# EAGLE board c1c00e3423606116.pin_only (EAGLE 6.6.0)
REV: D

Size 15.24 x 26.67 mm. Coordinates in mm from the lower left corner, seen from the top.
Outline: 15.24,25.4 15.24,2.29 14.48,1.52 11.18,1.52 9.65,0 2.54,0 0.76,1.78 0,1.78 0,25.4 arc-90 1.27,26.67 4.9,26.67 5.11,26.39 10.16,26.39 10.34,26.67 13.97,26.67 arc-90 15.24,25.4
Copper layers (1*16): Top 0.035mm / dielectric 1.5mm / Bottom 0.035mm
Design rules "adafruit": minimum track width 8mil, minimum drill 15.5mil, track to track 8mil, track to pad 8mil, pad to pad 8mil, via to via 8mil, smd to smd 8mil, copper to edge 10mil, drill to drill 8mil, minimum pad ring 10mil, minimum via ring 8mil, stop-mask expansion 2mil, vias tented up to drill 20mil, thermal gap 10mil
Net classes: 1 power: width 0.305 mm
Holes 2.2 mm at 1.52,20.19 13.72,20.19

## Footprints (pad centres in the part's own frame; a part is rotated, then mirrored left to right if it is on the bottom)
CHIPLED_0805_NOOUTLINE = smd 1.2 x 1.2: A 0,-1.05; C 0,1.05
JSTPH2 = smd 1 x 4.6: 1 -1,-3.7; 2 1,-3.7 | smd 1.6 x 3.4: NC1 -3.4,1.5; NC2 3.4,1.5
0805-NO = smd 1.3 x 1.5: 1 -0.95,0; 2 0.95,0
4UCONN_20329 = smd 1 x 2: BASE@1 -0.75,-2; BASE@2 0.75,-2 | smd 0.4 x 1.35: D+ 0,0.775; D- -0.65,0.775; GND 1.3,0.775; ID 0.65,0.775; VBUS -1.3,0.775 | drill 0.7 offset: SPRT@1 -3.3,0.9; SPRT@2 3.3,0.9 | drill 0.6 pad 2.5 square: SPRT@3 -3.6,-1.9; SPRT@4 3.6,-1.9 | hole 0.7: -1.95,0; 1.95,0
1X04-CLEANBIG = drill 1.016 pad 1.778: 1 -3.81,0; 2 -1.27,0; 3 1.27,0; 4 3.81,0
SOD-323 = smd 1.35 x 0.8: A 1.27,0; C -1.27,0
SOD-123FL = smd 0.91 x 1.22: A 1.637,0; C -1.637,0
SOT23-5L = smd 0.55 x 1.2: 1 -0.95,-1.3; 2 0,-1.3; 3 0.95,-1.3; 4 0.95,1.3; 5 -0.95,1.3
1X01-CLEANBIG = drill 1.016 pad 1.778: 1 0,0
BTN_KMR2_4.6X2.8 = smd 0.9 x 1: A 2.05,0.8; A' -2.05,0.8; B 2.05,-0.8; B' -2.05,-0.8
0603-NO = smd 1.1 x 1: 1 -0.85,0; 2 0.85,0
MLF20_4X4MM_0.5MM_ATMEL = smd 0.8 x 0.25: 1 -2,1; 2 -2,0.5; 3 -2,0; 4 -2,-0.5; 5 -2,-1; 11 2,-1; 12 2,-0.5; 13 2,0; 14 2,0.5; 15 2,1 | smd 0.25 x 0.8: 6 -1,-2; 7 -0.5,-2; 8 0,-2; 9 0.5,-2; 10 1,-2; 16 1,2; 17 0.5,2; 18 0,2; 19 -0.5,2; 20 -1,2 | smd 2.6 x 2.6: THERMAL 0,0
FIDUCIAL_1MM = smd 1 x 1: 1 0,0
MOUNTINGHOLE_2.0_PLATED = drill 2.2 pad 3: P$1 0,0

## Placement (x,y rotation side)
B1  red  [CHIPLED_0805_NOOUTLINE]  13.72,24.26 0 top
BAT  JST-PH2  [JSTPH2]  7.62,23.11 0 bottom
C1  10uF  [0805-NO]  4.32,17.91 90 top
C8  10uF  [0805-NO]  10.41,3.68 270 top
CN1  microUSB  [4UCONN_20329]  7.62,22.35 180 top
CN3  1X4-CLEANBIG  [1X04-CLEANBIG]  1.27,11.43 90 top
CN4  1X4-CLEANBIG  [1X04-CLEANBIG]  13.97,11.43 90 top
D1  3.6V  [SOD-323]  6.1,18.03 270 top
D2  SCHOTTKY  [SOD-123FL]  10.79,18.11 90 top
D3  3.6V  [SOD-323]  9.07,13.46 270 top
IC2  MIC5225-5.0v  [SOT23-5L]  6.07,13.34 270 top
JP1  [1X01-CLEANBIG]  13.97,17.78 0 top
JP2  [1X01-CLEANBIG]  1.27,17.78 0 top
PWR  green  [CHIPLED_0805_NOOUTLINE]  1.52,24.26 180 top
Q1  reset  [BTN_KMR2_4.6X2.8]  6.73,3.18 0 top
R1  68 (0603)  [0603-NO]  8.89,17.14 270 top
R2  68 (0603)  [0603-NO]  7.49,17.4 270 top
R3  1.5K (0603)  [0603-NO]  10.54,14.1 270 top
R4  470 (0603)  [0603-NO]  10.41,7.24 270 top
R5  470 (0603)  [0603-NO]  10.41,10.67 270 top
U1  ATtiny85-MU  [MLF20_4X4MM_0.5MM_ATMEL]  6.73,8.38 270 top
U$1  FIDUCIAL""  [FIDUCIAL_1MM]  9.14,19.81 0 top
U$5  [ADAFRUIT_3.5MM]  9.53,22.1 0 bottom
U$6  FIDUCIAL""  [FIDUCIAL_1MM]  7.3,3.18 0 top
U$8  MOUNTINGHOLE2.0  [MOUNTINGHOLE_2.0_PLATED]  1.91,3.81 0 top
U$9  MOUNTINGHOLE2.0  [MOUNTINGHOLE_2.0_PLATED]  13.34,3.81 0 top
U$12  [PCBFEAT-REV-040]  13.92,24.33 0 bottom
U$13  [SYMBOL_FCC_TINY]  12.74,13.67 0 bottom
U$14  [SYMBOL_CE_TINY]  6.52,13.67 0 bottom

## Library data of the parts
B1 BAT C1 C8 CN1 D1 D3 PWR Q1 R1-R5 U1 U$5 U$12-U$14 = microbuilder
CN3 CN4 D2 IC2 JP1 JP2 = adafruit
U$1 U$6 U$8 U$9 = microbuilder; BOM: EXCLUDE

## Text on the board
tPlace: PWR | #1 | BAT | USB | Gnd | #0 | #4 | #1 | #3 | #2 | Rst | 5V | Trinket 5v
bPlace: VBat | + | - | 5V logic | Vbat:5-16VDC / 150mA max / from 3V out | #3,#4 shared / with USB | Trinket | adafruit!

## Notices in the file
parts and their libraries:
microbuilder: This work is placed in the public domain, and may be freely used for commercial and non-commercial work with the following conditions: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
